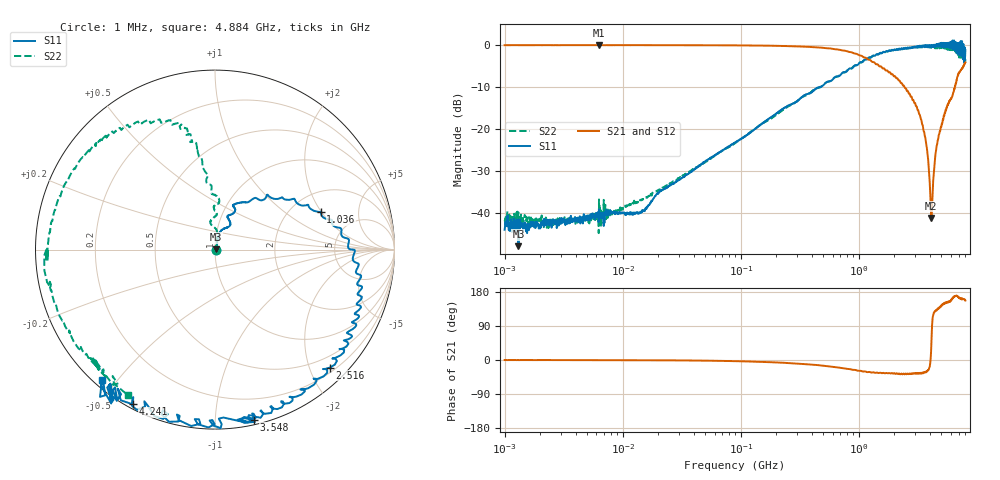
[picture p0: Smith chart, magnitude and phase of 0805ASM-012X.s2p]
!s-Parameter Generated by FASTRON Sdn. Bhd.
!FASTRON P/N : 0805ASM-012X
!Keysight Technologies: E5071C_MY46733604_B.14.02
!Date: Fri Jun 19 14:47:38 2026
!Version  :Rev00  Fri Jun 19 14:47:38 2026
!Data & Calibration Information:
!Freq  S11:SOLT2(ON)  S21:SOLT2(ON)  S12:SOLT2(ON)  S22:SOLT2(ON)
!PortZ  Port1:50+j0  Port2:50+j0
!When reading reference impedance value at option line is always used.
! Remarks : This data is being provided solely for informational purposes.
# Hz S dB R 50
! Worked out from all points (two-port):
!   1601 points, 1 MHz to 8 GHz, reference 50 ohm
!   highest |S21| = -0.04 dB at 6.301 MHz (marker M1); lowest = -41.1 dB at 4.116 GHz (marker M2)
!   |S21| within 3 dB of the highest: start of sweep to 1.133 GHz
!   lowest |S11| = -47.8 dB at 1.31 MHz (marker M3), VSWR 1.01, Z = 50.3 + j0.223 ohm
!   |S11| at or under -10 dB: start of sweep to 469.5 MHz
!   |S22| runs from -44.7 to -0.4 dB; largest |S21 - S12| = 0.016
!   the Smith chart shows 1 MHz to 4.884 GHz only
!   S11 on the Smith chart (normalised r, x): 1 MHz: 1.01, -0.00; 1.036 GHz: 2.88, +1.96; 2.516 GHz: 0.28, -2.34; 3.548 GHz: 0.04, -1.25; 4.241 GHz: 0.02, -0.60; 4.884 GHz: 0.03, -0.46
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1000000  -43.90 -7.0  -0.08 -0.1  -0.07 -0.1  -41.60 -1.3
1310238  -47.80 33.0  -0.11 0.1  -0.09 -0.1  -39.80 -12.4
4479405  -41.60 19.1  -0.08 -0.2  -0.08 -0.2  -41.90 22.9
6301378  -39.00 29.2  -0.04 -0.4  -0.04 -0.2  -36.70 35.5
1.414737e7  -39.60 51.9  -0.07 -0.6  -0.09 -0.6  -36.80 47.6
2.00676e7  -35.10 57.8  -0.08 -0.8  -0.09 -0.7  -34.50 61.9
8.994653e7  -23.20 75.3  -0.12 -3.1  -0.13 -3.1  -23.30 79.9
4.006501e8  -11.20 66.7  -0.52 -12.3  -0.53 -12.3  -11.00 85.3
1.035959e9  -4.09 19.4  -2.55 -28.6  -2.56 -28.7  -4.23 102.0
1.7949e9  -1.39 -17.7  -6.55 -34.3  -6.56 -34.7  -1.41 126.0
2.516241e9  -0.75 -45.8  -10.40 -37.0  -10.50 -37.1  -0.91 150.0
3.548043e9  -0.25 -77.1  -20.50 -32.6  -20.50 -32.5  -0.55 -180.0
3.791269e9  -0.20 -95.6  -25.00 -30.3  -25.00 -30.6  -0.51 -162.0
4.115571e9  -0.61 -115.0  -41.10 41.3  -41.10 40.8  -0.62 -143.0
4.240668e9  -0.21 -118.0  -34.00 115.0  -34.00 115.0  -0.70 -141.0
4.520586e9  -0.21 -126.0  -25.00 132.0  -25.00 132.0  -0.85 -137.0
4.88448e9  -0.36 -131.0  -20.50 139.0  -20.40 139.0  -0.49 -121.0
5.472309e9  -0.48 -154.0  -15.60 150.0  -15.50 150.0  -0.70 -77.3
5.918038e9  0.62 -155.0  -13.10 156.0  -13.10 155.0  -0.99 -72.9
6.534915e9  0.33 -162.0  -9.75 169.0  -9.77 168.0  -0.95 -25.6
7.306013e9  0.90 166.0  -6.00 162.0  -5.87 162.0  -2.21 -9.1
8e9  -1.22 133.0  -4.18 157.0  -4.08 156.0  -3.35 30.2
